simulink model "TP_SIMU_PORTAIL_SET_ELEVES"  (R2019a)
settings: Solver=VariableStepAuto  StartTime=0.0  StopTime=25  RelTol=1e-3
undefined symbols (not defined in the file): deg, kg, m, N, s
libraries: mblibv1 x17, fl_lib x13, nesl_utility x8, ee_lib x2, sdl_lib x1

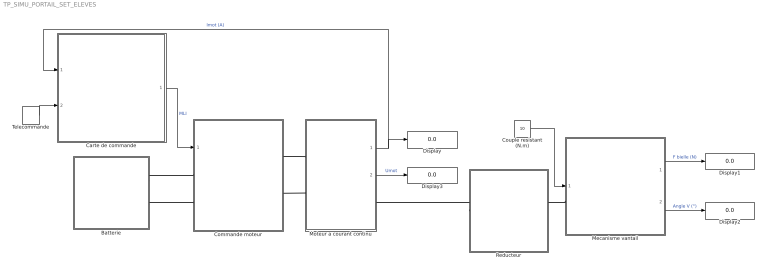
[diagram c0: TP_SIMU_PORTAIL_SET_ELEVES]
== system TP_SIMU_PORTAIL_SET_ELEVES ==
  Batterie : Subsystem
  Carte de commande : Stateflow chart  TreatAsAtomicUnit=on
  Commande moteur : Subsystem
  Couple resistant (N.m) : Constant  Value=10
  Display{,1..3} (4 alike) : Display
  Mecanisme vantail : Subsystem
  Moteur a courant continu : Subsystem
  Reducteur : Subsystem  mask{rend=1}
      mask prompts: rend "Rendement réducteur"
  Telecommande : DiscretePulseGenerator  PulseType=Time based  Period=30  PulseWidth=5
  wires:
  Moteur a courant continu/2(Umot) -> Display3/1  "Umot"
  Mecanisme vantail/1(Effort bielle) -> Display1/1  "F bielle (N)"
  Mecanisme vantail/2(Angle vantail) -> Display2/1  "Angle V (°)"
  Moteur a courant continu/1(Imot) -> Display/1, Carte de commande/1(imot)  "Imot (A)"
  Couple resistant (N.m)/1 -> Mecanisme vantail/1(Couple résistant)
  Telecommande/1 -> Carte de commande/2(bp)
  Carte de commande/1(reg) -> Commande moteur/1(Rapport cyclique)  "MLI"
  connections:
  Reducteur/RConn1 -- Mecanisme vantail/LConn1
  Reducteur/LConn1 -- Moteur a courant continu/RConn1
  Commande moteur/RConn1 -- Moteur a courant continu/LConn1
  Commande moteur/RConn2 -- Moteur a courant continu/LConn2
  Batterie/RConn1 -- Commande moteur/LConn1
  Batterie/RConn2 -- Commande moteur/LConn2

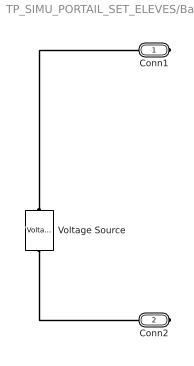
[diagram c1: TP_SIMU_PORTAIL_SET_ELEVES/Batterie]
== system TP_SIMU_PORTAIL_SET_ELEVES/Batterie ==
  Voltage Source : ee_lib/Sources/Voltage Source  dc_voltage=12 V  ac_voltage=0 V  ac_shift=0 rad  ac_frequency=60 Hz  noise_mode=0  PSD=0 V^2/Hz  repeatability=1  auto_seed=1935061431  user_seed=0  sample_time=1e-3 s  i_specify=off  i_priority=None  i=0 A  i_nominal_specify=off  i_nominal_unit=A  i_nominal_value=1  v_specify=off  v_priority=None  v=0 V  v_nominal_specify=off  v_nominal_unit=V  v_nominal_value=1
  Conn1 : PMIOPort  Side=Right
  Conn2 : PMIOPort  Port=2  Side=Right
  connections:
  Voltage Source/LConn1 -- Conn1/RConn1
  Voltage Source/RConn1 -- Conn2/RConn1

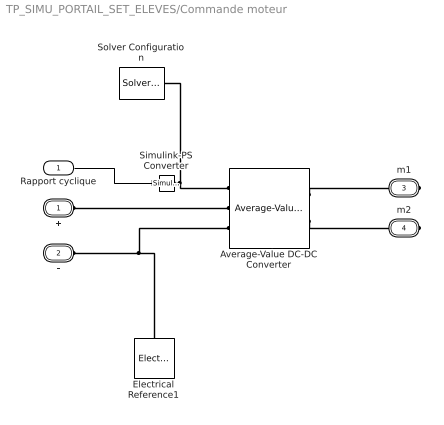
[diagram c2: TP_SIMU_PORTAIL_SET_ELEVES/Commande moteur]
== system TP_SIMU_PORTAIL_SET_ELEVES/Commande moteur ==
  Rapport cyclique : Inport
  Average-Value DC-DC Converter : ee_lib/Semiconductors & Converters/Converters/Average-Value DC-DC Converter  converter_type=1
  Electrical Reference1 : fl_lib/Electrical/Electrical Elements/Electrical Reference
  Simulink-PS Converter : nesl_utility/Simulink-PS Converter  PhysicalDomain=network_engine_domain  SubClassName=ps_input  LeftPortType=input  RightPortType=output  PseudoPeriodic=off  Frequencies=[]  NoiseDistribution=none  NoiseParameters=[]  Unit=1  AffineConversion=off  FilteringAndDerivatives=provide  SimscapeFilterOrder=1  InputFilterTimeConstant=0.001  UdotUserProvided=0
  Solver Configuration : nesl_utility/Solver Configuration  PhysicalDomain=network_engine_domain  SubClassName=solver  LeftPortType=input  RightPortType=generic  Tones=[]  Harmonics=[]  SimulateNoise=off  Profile=off  UseLocalSampling=off  EnableSwitchedLinearOptims=on  FrequencyDomain=off  UseCCode=off  RelTol=0.001  AbsTol=1e-06  MinStep=1e-09  ToWorkspace=off  RevertToSquareIcSolve=off  NumHomotopyIterations=100  PhasorMode=off  PhasorModeNumHarmonics=1  DoDC=off  ResidualTolerance=1e-9  UseLocalSolver=off  LocalSolverChoice=NE_BACKWARD_EULER_ADVANCER  LocalSolverSampleTime=.001  DoFixedCost=off  MaxNonlinIter=3  MaxModeIter=2  LinearAlgebra=Sparse  EquationFormulation=NE_TIME_EF  DelaysMemoryBudget=1024  AutomaticFiltering=on  FilteringTimeConstant=0.001  PartitionStorageMethod=AS_NEEDED  PartitionMemoryBudget=1024  PartitionMethod=FAST
  + : PMIOPort  Tag=PMCPort  Side=Left
  - : PMIOPort  Tag=PMCPort  Port=2  Side=Left
  m1 : PMIOPort  Tag=PMCPort  Port=3  Side=Right
  m2 : PMIOPort  Tag=PMCPort  Port=4  Side=Right
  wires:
  Rapport cyclique/1 -> Simulink-PS Converter/1
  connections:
  Average-Value DC-DC Converter/RConn1 -- m1/RConn1
  Average-Value DC-DC Converter/RConn2 -- m2/RConn1
  +/RConn1 -- Average-Value DC-DC Converter/LConn2
  -/RConn1 -- Electrical Reference1/LConn1 -- Average-Value DC-DC Converter/LConn3
  Simulink-PS Converter/RConn1 -- Solver Configuration/RConn1 -- Average-Value DC-DC Converter/LConn1

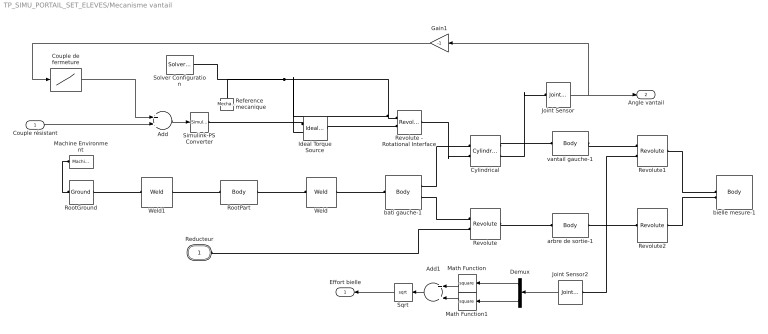
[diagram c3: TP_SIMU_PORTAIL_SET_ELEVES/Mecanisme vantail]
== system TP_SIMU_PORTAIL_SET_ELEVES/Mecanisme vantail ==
  Couple résistant : Inport
  Add : Sum
  Add1 : Sum
  Couple de fermeture : Lookup  InputValues=[0 89 90 90.1 90.2 90.3 100]  Table=[0 0 500 600 1000 2000 2000]
  Cylindrical : mblibv1/Joints/Cylindrical  LConnTagsString=__newl0|SA1  RConnTagsString=__newr0|SA1  UpdateFromCAD=on  NumSAPorts=2  CutJoint=off  MarkAsCut=off  Primitives=prismatic  PrimitiveProps=P1$World$[0,-1,0]$prismatic#R1$World$[0,-1,0]$revolute  DialogClass=JointBlock  P1Axis=[0,-1,0]  R1Axis=[0,-1,0]
  Demux : Demux  Outputs=3
  Gain1 : Gain  Gain=-1
  Ideal Torque Source : fl_lib/Mechanical/Mechanical Sources/Ideal Torque Source
  Joint Sensor : mblibv1/Sensors &  Actuators/Joint Sensor  UpdateFromCAD=off  PhysicalDomain=Mechanical  PortType=blob  Muxed=on  Pose=off  Angle=on  AngleUnits=deg  ArcVelocity=off  ArcVelocityUnits=deg/s  ArcAcceleration=off  ArcAccelerationUnits=deg/s^2  CoordPosition=on  CoordPositionUnits=m  Velocity=off  VelocityUnits=m/s  Acceleration=off  AccelerationUnits=m/s^2  Quaternion=on  QuaternionDT=off  QuaternionDDT=off  QuaternionUnits=off  OutputVector=[1]  ActiveIO=on  Width=1  DialogClass=MechanicalSensorBlock  Primitive=R1  Force=off  ForceUnits=N  Torque=off  TorqueUnits=N*m  ReferenceFrame=Absolute (World)  ReactionSensedSide=Base  ReactionReferenceFrame=Absolute (World)  ReactionForce=off  ReactionForceUnits=N  ReactionMoment=off  ReactionMomentUnits=N*m
  Joint Sensor2 : mblibv1/Sensors &  Actuators/Joint Sensor  UpdateFromCAD=off  PhysicalDomain=Mechanical  PortType=blob  Muxed=off  Pose=off  Angle=off  AngleUnits=deg  ArcVelocity=off  ArcVelocityUnits=deg/s  ArcAcceleration=off  ArcAccelerationUnits=deg/s^2  CoordPosition=on  CoordPositionUnits=m  Velocity=off  VelocityUnits=m/s  Acceleration=off  AccelerationUnits=m/s^2  Quaternion=on  QuaternionDT=off  QuaternionDDT=off  QuaternionUnits=off  OutputVector=[1]  ActiveIO=on  Width=3  DialogClass=MechanicalSensorBlock  Primitive=R1  Force=off  ForceUnits=N  Torque=off  TorqueUnits=N*m  ReferenceFrame=Absolute (World)  ReactionSensedSide=Base  ReactionReferenceFrame=Local (Body CS)  ReactionForce=on  ReactionForceUnits=N  ReactionMoment=off  ReactionMomentUnits=N*m
  Machine Environment : mblibv1/Bodies/Machine Environment  PortType=env  PhysicalDomain=Mechanical  DialogTemplateClass=MECH.MachineEnvironment  SyncWhenCopied=off  Gravity=[0 -9.81 0]  GravityUnits=m/s^2  GravityAsSignal=off  Dimensionality=Auto-detect  AnalysisType=Forward dynamics  LinearAssemblyTolerance=1e-3  LinearAssemblyToleranceUnits=m  AngularAssemblyTolerance=1e-3  AngularAssemblyToleranceUnits=rad  ConstraintSolverType=Stabilizing  ConstraintRelTolerance=1e-4  ConstraintAbsTolerance=1e-4  UseRobustSingularityHandling=off  RedundancyAnalysisToleranceType=Automatically select tolerance  RedundancyAnalysisTolerance=1e-14  StatePerturbationType=Fixed  PerturbationSize=1e-5  VisualizeMachine=on  BodyVisualizationType=Use model default body geometries  BodyColorSelMode=Use model default  DefaultBodyColor=[1 0 0]
  Math Function : Math  Operator=square
  Math Function1 : Math  Operator=square
  Reference mecanique : fl_lib/Mechanical/Rotational Elements/Mechanical Rotational Reference
  Revolute : mblibv1/Joints/Revolute  LConnTagsString=__newl0|SA1  RConnTagsString=__newr0  UpdateFromCAD=on  NumSAPorts=1  CutJoint=off  MarkAsCut=off  Primitives=prismatic  PrimitiveProps=R1$World$[0,-1,0]$revolute  DialogClass=JointBlock  R1Axis=[0,-1,0]
  Revolute - Rotational Interface : mblibv1/Interface  Elements/Revolute - Rotational Interface  UpdateFromCAD=off  DialogClass=RevoluteRotationalInterface  Primitive=R1  InputFiltering=off  SimscapeFilterOrder=1  InputFilterTimeConstant=0.001
  Revolute1 : mblibv1/Joints/Revolute  LConnTagsString=__newl0|SA1  RConnTagsString=__newr0  UpdateFromCAD=on  NumSAPorts=1  CutJoint=off  MarkAsCut=off  Primitives=prismatic  PrimitiveProps=R1$World$[0,-1,0]$revolute  DialogClass=JointBlock  R1Axis=[0,-1,0]
  Revolute2 : mblibv1/Joints/Revolute  LConnTagsString=__newl0  RConnTagsString=__newr0  UpdateFromCAD=on  NumSAPorts=0  CutJoint=off  MarkAsCut=off  Primitives=prismatic  PrimitiveProps=R1$World$[0,1,0]$revolute  DialogClass=JointBlock  R1Axis=[0,1,0]
  RootGround : mblibv1/Bodies/Ground  UpdateFromCAD=on  LeftPortType=env  RightPortType=workingframe  PhysicalDomain=Mechanical  DialogClass=GroundBlock  CoordPosition=[-0.151407,0.157148,0.314075]  CoordPositionUnits=m  StateVectorMgrId=-1  MachineId=[0 0]  ShowEnvPort=on  ParameterChecksum=[3723735524, 4162897784, 1326464849, 2568284377]  TopologyChecksum=[2672908821, 872372531, 2603072148, 984099915]
  RootPart : mblibv1/Bodies/Body  LConnTagsString=CS3  RConnTagsString=CS2  UpdateFromCAD=on  DialogClass=MechanicalBodyBlock  Mass=0  MassUnits=kg  InertiaUnits=kg*m^2  Inertia=[0,0,0;0,0,0;0,0,0]  Shape=Cylinder  ShapeDims=[1 1]  ShapeUnits=m  ShapeUse=false  Density=1  DensityUnits=kg/m^3  DensityUse=false  GraphicsMode=MACHINE_DEFAULT  BodyColorSelMode=MACHINE_DEFAULT  BodyColor=[1;0;0]  AttachedToCS=CS1  CG=Right$CG$[-0.151407 0.157148 0.314075]$WORLD$WORLD$m$[1 0 0;0 1 0;0 0 1]$3x3 Transform$rad$WORLD$false$none  WorkingFrames=Right$CS1$[0 0 0]$WORLD$WORLD$m$[1 0 0;0 1 0;0 0 1]$3x3 Transform$rad$WORLD$false$none#Right$CS2$[-0.154192 0.157154 0.312848]$WORLD$WORLD$m$[1 0 0;0 1 0;0 0 1]$3x3 Transform$rad$WORLD$true$none#Left$CS3$[-0.151407 0.157148 0.314075]$WORLD$WORLD$m$[1 0 0;0 1 0;0 0 1]$3x3 Transform$rad$WORLD$true$none  CGPos=[-0.151407 0.157148 0.314075]  CGRot=[1 0 0;0 1 0;0 0 1]  CS0Pos=[]  CS0Rot=[]  CS1Pos=[0 0 0]  CS1Rot=[1 0 0;0 1 0;0 0 1]  CS2Pos=[-0.154192 0.157154 0.312848]  CS2Rot=[1 0 0;0 1 0;0 0 1]  CS3Pos=[-0.151407 0.157148 0.314075]  CS3Rot=[1 0 0;0 1 0;0 0 1]  CS4Pos=[]  CS4Rot=[]  CS5Pos=[]  CS5Rot=[]  CS6Pos=[]  CS6Rot=[]  CS7Pos=[]  CS7Rot=[]  CS8Pos=[]  CS8Rot=[]  CS9Pos=[]  CS9Rot=[]  CS10Pos=[]  CS10Rot=[]  CS11Pos=[]  CS11Rot=[]  CS12Pos=[]  CS12Rot=[]  CS13Pos=[]  CS13Rot=[]  CS14Pos=[]  CS14Rot=[]  CS15Pos=[]  CS15Rot=[]  CS16Pos=[]  CS16Rot=[]  CS17Pos=[]  CS17Rot=[]  CS18Pos=[]  CS18Rot=[]  CS19Pos=[]  CS19Rot=[]  CS20Pos=[]  CS20Rot=[]
  Simulink-PS Converter : nesl_utility/Simulink-PS Converter  PhysicalDomain=network_engine_domain  SubClassName=ps_input  LeftPortType=input  RightPortType=output  PseudoPeriodic=off  Frequencies=[]  NoiseDistribution=none  NoiseParameters=[]  Unit=N*m  AffineConversion=off  FilteringAndDerivatives=filter  SimscapeFilterOrder=1  InputFilterTimeConstant=.001  UdotUserProvided=1
  Solver Configuration : nesl_utility/Solver Configuration  PhysicalDomain=network_engine_domain  SubClassName=solver  LeftPortType=input  RightPortType=generic  Tones=[]  Harmonics=[]  SimulateNoise=off  Profile=off  UseLocalSampling=off  EnableSwitchedLinearOptims=on  FrequencyDomain=off  UseCCode=off  RelTol=0.001  AbsTol=1e-06  MinStep=1e-09  ToWorkspace=off  RevertToSquareIcSolve=off  NumHomotopyIterations=100  PhasorMode=off  PhasorModeNumHarmonics=1  DoDC=off  ResidualTolerance=1e-09  UseLocalSolver=off  LocalSolverChoice=NE_BACKWARD_EULER_ADVANCER  LocalSolverSampleTime=0.001  DoFixedCost=off  MaxNonlinIter=3  MaxModeIter=2  LinearAlgebra=auto  EquationFormulation=NE_TIME_EF  DelaysMemoryBudget=1024  AutomaticFiltering=on  FilteringTimeConstant=0.001  PartitionStorageMethod=AS_NEEDED  PartitionMemoryBudget=1024  PartitionMethod=ROBUST
  Sqrt : Sqrt
  Weld : mblibv1/Joints/Weld  LConnTagsString=__newl0  RConnTagsString=__newr0  UpdateFromCAD=on  NumSAPorts=0  CutJoint=off  MarkAsCut=off  Primitives=weld  PrimitiveProps=W$WORLD$[0.57735,0.57735,0.57735]$weld  DialogClass=JointBlock  WAxis=[0.57735,0.57735,0.57735]
  Weld1 : mblibv1/Joints/Weld  LConnTagsString=__newl0  RConnTagsString=__newr0  UpdateFromCAD=on  NumSAPorts=0  CutJoint=off  MarkAsCut=off  Primitives=weld  PrimitiveProps=W$WORLD$[0.57735,0.57735,0.57735]$weld  DialogClass=JointBlock  WAxis=[0.57735,0.57735,0.57735]
  arbre de sortie-1 : mblibv1/Bodies/Body  LConnTagsString=CS2  RConnTagsString=CS3  UpdateFromCAD=on  DialogClass=MechanicalBodyBlock  Mass=0.30162  MassUnits=kg  InertiaUnits=kg*m^2  Inertia=[0.00644566,-7.6265e-08,8.94984e-06;-7.6265e-08,0.00635041,-3.14078e-06;8.94984e-06,-3.14078e-06,0.000124114]  Shape=Cylinder  ShapeDims=[1 1]  ShapeUnits=m  ShapeUse=false  Density=1  DensityUnits=kg/m^3  DensityUse=false  GraphicsMode=GFXFILE  GraphicsFileName=SET-simulink - arbre de sortie-1.STL  BodyColorSelMode=COLORPALETTE  BodyColor=[1;0;0]  AttachedToCS=CS1  CG=Right$CG$[-0.193258 0.0428945 0.377026]$WORLD$WORLD$m$[0 -0.562668 0.826683;-1 0 0;0 -0.826683 -0.562668]$3x3 Transform$rad$WORLD$false$none  WorkingFrames=Right$CS1$[-0.0610122 0.0964541 0.336929]$WORLD$WORLD$m$[0 -0.562668 0.826683;-1 0 0;0 -0.826683 -0.562668]$3x3 Transform$rad$WORLD$false$none#Left$CS2$[-0.0777712 0.0617 0.298506]$WORLD$WORLD$m$[1 0 0;0 1 0;0 0 1]$3x3 Transform$rad$WORLD$true$none#Right$CS3$[-0.408444 0.0337 0.523573]$WORLD$WORLD$m$[1 0 0;0 1 0;0 0 1]$3x3 Transform$rad$WORLD$true$none  CGPos=[-0.193258 0.0428945 0.377026]  CGRot=[0 -0.562668 0.826683;-1 0 0;0 -0.826683 -0.562668]  CS0Pos=[]  CS0Rot=[]  CS1Pos=[-0.0610122 0.0964541 0.336929]  CS1Rot=[0 -0.562668 0.826683;-1 0 0;0 -0.826683 -0.562668]  CS2Pos=[-0.0777712 0.0617 0.298506]  CS2Rot=[1 0 0;0 1 0;0 0 1]  CS3Pos=[-0.408444 0.0337 0.523573]  CS3Rot=[1 0 0;0 1 0;0 0 1]  CS4Pos=[]  CS4Rot=[]  CS5Pos=[]  CS5Rot=[]  CS6Pos=[]  CS6Rot=[]  CS7Pos=[]  CS7Rot=[]  CS8Pos=[]  CS8Rot=[]  CS9Pos=[]  CS9Rot=[]  CS10Pos=[]  CS10Rot=[]  CS11Pos=[]  CS11Rot=[]  CS12Pos=[]  CS12Rot=[]  CS13Pos=[]  CS13Rot=[]  CS14Pos=[]  CS14Rot=[]  CS15Pos=[]  CS15Rot=[]  CS16Pos=[]  CS16Rot=[]  CS17Pos=[]  CS17Rot=[]  CS18Pos=[]  CS18Rot=[]  CS19Pos=[]  CS19Rot=[]  CS20Pos=[]  CS20Rot=[]
  bati gauche-1 : mblibv1/Bodies/Body  LConnTagsString=CS2  RConnTagsString=CS3|CS4  UpdateFromCAD=on  DialogClass=MechanicalBodyBlock  Mass=64.0295  MassUnits=kg  InertiaUnits=kg*m^2  Inertia=[0.698446,0.0155862,0.05942;0.0155862,0.732189,0.097542;0.05942,0.097542,0.797231]  Shape=Cylinder  ShapeDims=[1 1]  ShapeUnits=m  ShapeUse=false  Density=1  DensityUnits=kg/m^3  DensityUse=false  GraphicsMode=GFXFILE  GraphicsFileName=SET-simulink - bati gauche-1.STL  BodyColorSelMode=COLORPALETTE  BodyColor=[0.752941;0.752941;0.752941]  AttachedToCS=CS1  CG=Right$CG$[-0.154192 0.157154 0.312848]$WORLD$WORLD$m$[1 0 0;0 1 0;0 0 1]$3x3 Transform$rad$WORLD$false$none  WorkingFrames=Right$CS1$[0 0 0]$WORLD$WORLD$m$[1 0 0;0 1 0;0 0 1]$3x3 Transform$rad$WORLD$false$none#Left$CS2$[-0.154192 0.157154 0.312848]$WORLD$WORLD$m$[1 0 0;0 1 0;0 0 1]$3x3 Transform$rad$WORLD$true$none#Right$CS3$[0.0192288 0.466 0.02]$WORLD$WORLD$m$[1 0 0;0 1 0;0 0 1]$3x3 Transform$rad$WORLD$true$none#Right$CS4$[-0.0777712 0.0617 0.298506]$WORLD$WORLD$m$[1 0 0;0 1 0;0 0 1]$3x3 Transform$rad$WORLD$true$non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  CGPos=[-0.154192 0.157154 0.312848]  CGRot=[1 0 0;0 1 0;0 0 1]  CS0Pos=[]  CS0Rot=[]  CS1Pos=[0 0 0]  CS1Rot=[1 0 0;0 1 0;0 0 1]  CS2Pos=[-0.154192 0.157154 0.312848]  CS2Rot=[1 0 0;0 1 0;0 0 1]  CS3Pos=[0.0192288 0.466 0.02]  CS3Rot=[1 0 0;0 1 0;0 0 1]  CS4Pos=[-0.0777712 0.0617 0.298506]  CS4Rot=[1 0 0;0 1 0;0 0 1]  CS5Pos=[]  CS5Rot=[]  CS6Pos=[]  CS6Rot=[]  CS7Pos=[]  CS7Rot=[]  CS8Pos=[]  CS8Rot=[]  CS9Pos=[]  CS9Rot=[]  CS10Pos=[]  CS10Rot=[]  CS11Pos=[]  CS11Rot=[]  CS12Pos=[]  CS12Rot=[]  CS13Pos=[]  CS13Rot=[]  CS14Pos=[]  CS14Rot=[]  CS15Pos=[]  CS15Rot=[]  CS16Pos=[]  CS16Rot=[]  CS17Pos=[]  CS17Rot=[]  CS18Pos=[]  CS18Rot=[]  CS19Pos=[]  CS19Rot=[]  CS20Pos=[]  CS20Rot=[]
  bielle mesure-1 : mblibv1/Bodies/Body  LConnTagsString=CS2|CS3  UpdateFromCAD=on  DialogClass=MechanicalBodyBlock  Mass=0.193239  MassUnits=kg  InertiaUnits=kg*m^2  Inertia=[6.64886e-05,-1.89129e-06,1.037e-05;-1.89129e-06,0.00224291,-8.89446e-07;1.037e-05,-8.89446e-07,0.0022327]  Shape=Cylinder  ShapeDims=[1 1]  ShapeUnits=m  ShapeUse=false  Density=1  DensityUnits=kg/m^3  DensityUse=false  GraphicsMode=GFXFILE  GraphicsFileName=SET-simulink - bielle mesure-1.STL  BodyColorSelMode=COLORPALETTE  BodyColor=[0;1;1]  AttachedToCS=CS1  CG=Right$CG$[-0.220186 0.0682669 0.570415]$WORLD$WORLD$m$[-0.970807 -0.239862 0;0 0 1;-0.239862 0.970807 0]$3x3 Transform$rad$WORLD$false$none  WorkingFrames=Right$CS1$[-0.0901299 0.053 0.561371]$WORLD$WORLD$m$[-0.970807 -0.239862 0;0 0 1;-0.239862 0.970807 0]$3x3 Transform$rad$WORLD$false$none#Left$CS2$[-0.0317712 0.0635 0.61664]$WORLD$WORLD$m$[1 0 0;0 1 0;0 0 1]$3x3 Transform$rad$WORLD$true$none#Left$CS3$[-0.408444 0.0337 0.523573]$WORLD$WORLD$m$[1 0 0;0 1 0;0 0 1]$3x3 Transform$rad$WORLD$true$none  CGPos=[-0.220186 0.0682669 0.570415]  CGRot=[-0.970807 -0.239862 0;0 0 1;-0.239862 0.970807 0]  CS0Pos=[]  CS0Rot=[]  CS1Pos=[-0.0901299 0.053 0.561371]  CS1Rot=[-0.970807 -0.239862 0;0 0 1;-0.239862 0.970807 0]  CS2Pos=[-0.0317712 0.0635 0.61664]  CS2Rot=[1 0 0;0 1 0;0 0 1]  CS3Pos=[-0.408444 0.0337 0.523573]  CS3Rot=[1 0 0;0 1 0;0 0 1]  CS4Pos=[]  CS4Rot=[]  CS5Pos=[]  CS5Rot=[]  CS6Pos=[]  CS6Rot=[]  CS7Pos=[]  CS7Rot=[]  CS8Pos=[]  CS8Rot=[]  CS9Pos=[]  CS9Rot=[]  CS10Pos=[]  CS10Rot=[]  CS11Pos=[]  CS11Rot=[]  CS12Pos=[]  CS12Rot=[]  CS13Pos=[]  CS13Rot=[]  CS14Pos=[]  CS14Rot=[]  CS15Pos=[]  CS15Rot=[]  CS16Pos=[]  CS16Rot=[]  CS17Pos=[]  CS17Rot=[]  CS18Pos=[]  CS18Rot=[]  CS19Pos=[]  CS19Rot=[]  CS20Pos=[]  CS20Rot=[]
  vantail gauche-1 : mblibv1/Bodies/Body  LConnTagsString=CS2  RConnTagsString=CS3  UpdateFromCAD=on  DialogClass=MechanicalBodyBlock  Mass=1.19959  MassUnits=kg  InertiaUnits=kg*m^2  Inertia=[0.021331,0.00759461,-0.000142522;0.00759461,0.0455399,6.62125e-05;-0.000142522,6.62125e-05,0.0668166]  Shape=Cylinder  ShapeDims=[1 1]  ShapeUnits=m  ShapeUse=false  Density=1  DensityUnits=kg/m^3  DensityUse=false  GraphicsMode=GFXFILE  GraphicsFileName=SET-simulink - vantail gauche-1.STL  BodyColorSelMode=COLORPALETTE  BodyColor=[1;1;0]  AttachedToCS=CS1  CG=Right$CG$[0.018825 0.19986 0.32244]$WORLD$WORLD$m$[0 0 -1;0 1 0;1 0 0]$3x3 Transform$rad$WORLD$false$none  WorkingFrames=Right$CS1$[0.0237288 0.03824 0.04]$WORLD$WORLD$m$[0 0 -1;0 1 0;1 0 0]$3x3 Transform$rad$WORLD$false$none#Left$CS2$[0.0192288 0.466 0.02]$WORLD$WORLD$m$[1 0 0;0 1 0;0 0 1]$3x3 Transform$rad$WORLD$true$none#Right$CS3$[-0.0317712 0.0635 0.61664]$WORLD$WORLD$m$[1 0 0;0 1 0;0 0 1]$3x3 Transform$rad$WORLD$true$none  CGPos=[0.018825 0.19986 0.32244]  CGRot=[0 0 -1;0 1 0;1 0 0]  CS0Pos=[]  CS0Rot=[]  CS1Pos=[0.0237288 0.03824 0.04]  CS1Rot=[0 0 -1;0 1 0;1 0 0]  CS2Pos=[0.0192288 0.466 0.02]  CS2Rot=[1 0 0;0 1 0;0 0 1]  CS3Pos=[-0.0317712 0.0635 0.61664]  CS3Rot=[1 0 0;0 1 0;0 0 1]  CS4Pos=[]  CS4Rot=[]  CS5Pos=[]  CS5Rot=[]  CS6Pos=[]  CS6Rot=[]  CS7Pos=[]  CS7Rot=[]  CS8Pos=[]  CS8Rot=[]  CS9Pos=[]  CS9Rot=[]  CS10Pos=[]  CS10Rot=[]  CS11Pos=[]  CS11Rot=[]  CS12Pos=[]  CS12Rot=[]  CS13Pos=[]  CS13Rot=[]  CS14Pos=[]  CS14Rot=[]  CS15Pos=[]  CS15Rot=[]  CS16Pos=[]  CS16Rot=[]  CS17Pos=[]  CS17Rot=[]  CS18Pos=[]  CS18Rot=[]  CS19Pos=[]  CS19Rot=[]  CS20Pos=[]  CS20Rot=[]
  Reducteur : PMIOPort  Side=Left
  Effort bielle : Outport
  Angle vantail : Outport  Port=2
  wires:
  Gain1/1 -> Couple de fermeture/1
  Add/1 -> Simulink-PS Converter/1
  Joint Sensor2/1 -> Demux/1
  Demux/1 -> Math Function/1
  Demux/3 -> Math Function1/1
  Math Function/1 -> Add1/1
  Math Function1/1 -> Add1/2
  Add1/1 -> Sqrt/1
  Sqrt/1 -> Effort bielle/1
  Couple de fermeture/1 -> Add/1
  Joint Sensor/1 -> Angle vantail/1, Gain1/1
  Couple résistant/1 -> Add/2
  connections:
  RootPart/RConn1 -- Weld/LConn1
  Weld/RConn1 -- bati gauche-1/LConn1
  bati gauche-1/RConn1 -- Cylindrical/LConn1
  Cylindrical/RConn1 -- vantail gauche-1/LConn1
  bati gauche-1/RConn2 -- Revolute/LConn1
  vantail gauche-1/RConn1 -- Revolute1/LConn1
  Revolute/RConn1 -- arbre de sortie-1/LConn1
  arbre de sortie-1/RConn1 -- Revolute2/LConn1
  Revolute1/RConn1 -- bielle mesure-1/LConn1
  Revolute2/RConn1 -- bielle mesure-1/LConn2
  RootGround/RConn1 -- Weld1/LConn1
  Weld1/RConn1 -- RootPart/LConn1
  RootGround/LConn1 -- Machine Environment/RConn1
  Reducteur/RConn1 -- Revolute/LConn2
  Cylindrical/RConn2 -- Joint Sensor/LConn1
  Revolute - Rotational Interface/RConn1 -- Cylindrical/LConn2
  Joint Sensor2/LConn1 -- Revolute1/LConn2
  Revolute - Rotational Interface/LConn1 -- Solver Configuration/RConn1 -- Reference mecanique/LConn1 -- Ideal Torque Source/RConn2
  Ideal Torque Source/RConn1 -- Simulink-PS Converter/RConn1
  Ideal Torque Source/LConn1 -- Revolute - Rotational Interface/LConn2

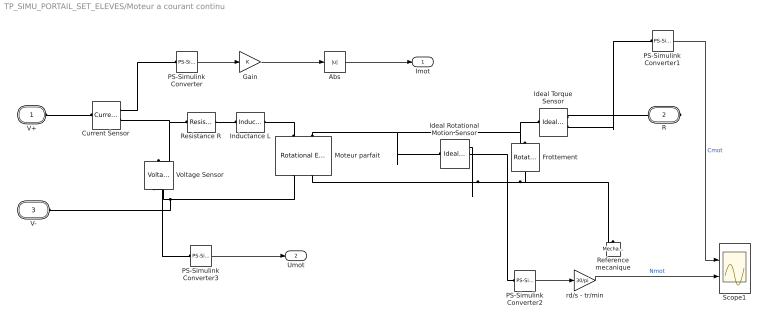
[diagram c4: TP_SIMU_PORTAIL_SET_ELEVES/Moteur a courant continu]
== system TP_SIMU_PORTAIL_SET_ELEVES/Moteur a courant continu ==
  Abs : Abs
  Current Sensor : fl_lib/Electrical/Electrical Sensors/Current Sensor
  Frottement : fl_lib/Mechanical/Rotational Elements/Rotational Friction  brkwy_trq=0.002 N*m  brkwy_vel=0.0082085 rad/s  Col_trq=0.002 N*m  visc_coef=5e-10 N*m/(rad/s)  w_specify=off  w_priority=None  w=0 rad/s  w_nominal_specify=off  w_nominal_unit=rad/s  w_nominal_value=1  t_specify=off  t_priority=None  t=0 N*m  t_nominal_specify=off  t_nominal_unit=N*m  t_nominal_value=1
  Gain : Gain
  Ideal Rotational Motion Sensor : fl_lib/Mechanical/Mechanical Sensors/Ideal Rotational Motion Sensor  offset=0 rad
  Ideal Torque Sensor : fl_lib/Mechanical/Mechanical Sensors/Ideal Torque Sensor
  Inductance L : fl_lib/Electrical/Electrical Elements/Inductor  l=0.1 mH  r=0 Ohm  g=1e-09 1/Ohm  i_specify=off  i_priority=None  i=0 A  i_nominal_specify=off  i_nominal_unit=A  i_nominal_value=1  v_specify=off  v_priority=None  v=0 V  v_nominal_specify=off  v_nominal_unit=V  v_nominal_value=1  i_L_specify=on  i_L_priority=High  i_L=0 A  i_L_nominal_specify=off  i_L_nominal_unit=A  i_L_nominal_value=1
  Moteur parfait : fl_lib/Electrical/Electrical Elements/Rotational Electromechanical Converter  K=0.0653 V/(rad/s)  i_specify=off  i_priority=None  i=0 A  i_nominal_specify=off  i_nominal_unit=A  i_nominal_value=1  v_specify=off  v_priority=None  v=0 V  v_nominal_specify=off  v_nominal_unit=V  v_nominal_value=1  t_specify=off  t_priority=None  t=0 N*m  t_nominal_specify=off  t_nominal_unit=N*m  t_nominal_value=1  w_specify=off  w_priority=None  w=0 rad/s  w_nominal_specify=off  w_nominal_unit=rad/s  w_nominal_value=1
  PS-Simulink Converter : nesl_utility/PS-Simulink Converter  PhysicalDomain=network_engine_domain  SubClassName=ps_output  LeftPortType=input  RightPortType=output  PseudoPeriodic=off  Frequencies=[]  Unit=A  AffineConversion=off
  PS-Simulink Converter1 : nesl_utility/PS-Simulink Converter  PhysicalDomain=network_engine_domain  SubClassName=ps_output  LeftPortType=input  RightPortType=output  PseudoPeriodic=off  Frequencies=[]  Unit=N*m  AffineConversion=off
  PS-Simulink Converter2 : nesl_utility/PS-Simulink Converter  PhysicalDomain=network_engine_domain  SubClassName=ps_output  LeftPortType=input  RightPortType=output  PseudoPeriodic=off  Frequencies=[]  Unit=rad/s  AffineConversion=off
  PS-Simulink Converter3 : nesl_utility/PS-Simulink Converter  PhysicalDomain=network_engine_domain  SubClassName=ps_output  LeftPortType=input  RightPortType=output  PseudoPeriodic=off  Frequencies=[]  Unit=V  AffineConversion=off
  Reference mecanique : fl_lib/Mechanical/Rotational Elements/Mechanical Rotational Reference
  Resistance R : fl_lib/Electrical/Electrical Elements/Resistor  Tag=Factory Generic  R=0.7 Ohm  i_specify=off  i_priority=None  i=0 A  i_nominal_specify=off  i_nominal_unit=A  i_nominal_value=1  v_specify=off  v_priority=None  v=0 V  v_nominal_specify=off  v_nominal_unit=V  v_nominal_value=1
  Scope1 : Scope  NumInputPorts=2
  Voltage Sensor : fl_lib/Electrical/Electrical Sensors/Voltage Sensor
  rd/s - tr/min : Gain  Gain=30/pi
  V+ : PMIOPort  Side=Left
  R : PMIOPort  Port=2  Side=Right
  V- : PMIOPort  Port=3  Side=Left
  Imot : Outport
  Umot : Outport  Port=2
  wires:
  PS-Simulink Converter/1 -> Gain/1
  Gain/1 -> Abs/1
  PS-Simulink Converter1/1 -> Scope1/1  "Cmot"
  PS-Simulink Converter2/1 -> rd/s - tr/min/1
  rd/s - tr/min/1 -> Scope1/2  "Nmot"
  PS-Simulink Converter3/1 -> Umot/1
  Abs/1 -> Imot/1
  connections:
  Moteur parfait/LConn1 -- Inductance L/RConn1
  Moteur parfait/RConn1 -- V-/RConn1 -- Voltage Sensor/RConn2
  Inductance L/LConn1 -- Resistance R/RConn1
  Moteur parfait/RConn2 -- Reference mecanique/LConn1 -- Frottement/RConn1 -- Ideal Rotational Motion Sensor/RConn1
  Current Sensor/LConn1 -- V+/RConn1
  Current Sensor/RConn1 -- PS-Simulink Converter/LConn1
  Moteur parfait/LConn2 -- Ideal Torque Sensor/LConn1 -- Frottement/LConn1 -- Ideal Rotational Motion Sensor/LConn1
  PS-Simulink Converter1/LConn1 -- Ideal Torque Sensor/RConn2
  Ideal Torque Sensor/RConn1 -- R/RConn1
  PS-Simulink Converter2/LConn1 -- Ideal Rotational Motion Sensor/RConn2
  Resistance R/LConn1 -- Current Sensor/RConn2 -- Voltage Sensor/LConn1
  PS-Simulink Converter3/LConn1 -- Voltage Sensor/RConn1

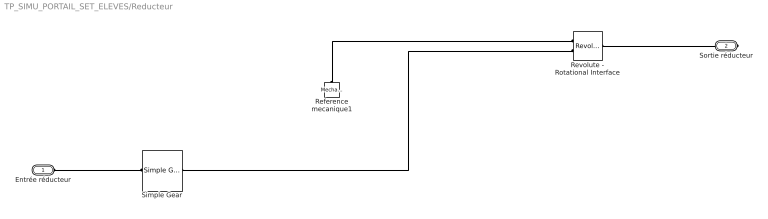
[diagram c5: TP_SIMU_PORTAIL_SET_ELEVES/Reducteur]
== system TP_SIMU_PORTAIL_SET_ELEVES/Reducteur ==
  Reference mecanique1 : fl_lib/Mechanical/Rotational Elements/Mechanical Rotational Reference
  Revolute - Rotational Interface : mblibv1/Interface  Elements/Revolute - Rotational Interface  UpdateFromCAD=off  DialogClass=RevoluteRotationalInterface  Primitive=R1  InputFiltering=off  SimscapeFilterOrder=1  InputFilterTimeConstant=0.001
  Simple Gear : sdl_lib/Gears/Simple Gear  ratio=1083  rotation_direction=2  friction_model=2  T_noload=0.1 N*m  T_nom=5 N*m  efficiency_nom=0.8  efficiency=rend  mu_visc=[ 0 0 ] N*m/(rad/s)  w_thr=0.01 rad/s  pwr_thr=0.001 W  enable_faults=simscape.enum.onoff.off  efficiency_fault=0.05  external_fault=simscape.enum.onoff.off  temporal_fault=simscape.enum.onoff.off  fault_time=5 s  fault_angles=pi / 12 rad  report_fault=1  temperature_TLU=[ 280 300 320 ] K  load_TLU=[ 1 5 10 ] N*m  efficiency_TLU=[ 0.95 0.9 0.85 ]  efficiency_TLU2=[ 0.85 0.8 0.75; 0.95 0.9 0.85; 0.85 0.8 0.7 ]  thermal_mass=50 J/K  T_init=300 K
  Entrée réducteur : PMIOPort  Side=Left
  Sortie réducteur : PMIOPort  Port=2  Side=Right
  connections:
  Sortie réducteur/RConn1 -- Revolute - Rotational Interface/RConn1
  Simple Gear/LConn1 -- Entrée réducteur/RConn1
  Revolute - Rotational Interface/LConn2 -- Simple Gear/RConn1
  Reference mecanique1/LConn1 -- Revolute - Rotational Interface/LConn1

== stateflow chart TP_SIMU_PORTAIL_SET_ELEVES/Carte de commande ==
  state ARRET
    reg=0;
  state PLEINE_VITESSE
    reg=1
  state VITESSE_REDUITE
    reg=0.28;
  (default) -> ARRET
  VITESSE_REDUITE -> ARRET : [imot>=4]
  ARRET -> PLEINE_VITESSE : [bp==1]
  PLEINE_VITESSE -> VITESSE_REDUITE : after(15,sec)
  data: reg output double; imot input; bp input
